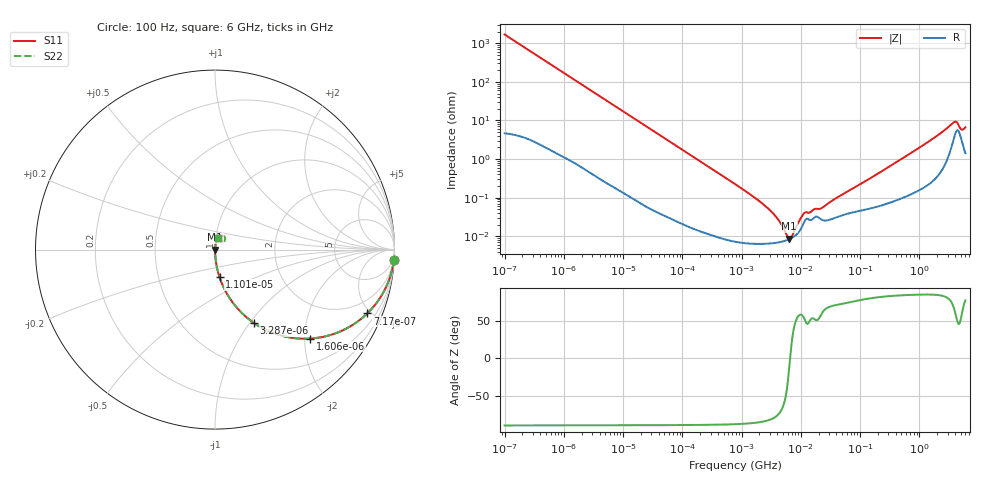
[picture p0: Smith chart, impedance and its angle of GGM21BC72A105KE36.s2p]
!Murata Part Number: GGM21BC72A105KE36
!These Parameters are Measured in Series Mode Connection
!Data Generated on Mar 13, 2026
!  o--ll--o
!Port1  Port2
!  o------o
!Operation Temp=25[degC], DC Bias Voltage=0[V]
!Freq. Start=100[Hz] Stop=6[GHz] 401[Steps]
# Hz S RI R 50
!Freq.(Hz) S11(Real) S11(Imag) S21(Real) S21(Imag) S12(Real) S12(Imag) S22(Real) S22(Imag)
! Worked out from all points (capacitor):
!   401 points, 100 Hz to 6 GHz, reference 50 ohm
!   read as one part in series: C = 938 nF near 109 Hz
!   lowest |Z| = 8.58 mohm at 6.353 MHz (marker M1)
!   series resonance near 6.592 MHz, so ESL is about 620 pH
!   S11 on the Smith chart (normalised r, x): 100 Hz: 1, -34; 717 Hz: 1.03, -4.76; 1.606 kHz: 1.01, -2.13; 3.287 kHz: 1.01, -1.05; 11.01 kHz: 1.00, -0.31; 6 GHz: 1.03, +0.13
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100  0.9964 -0.0588  0.00363 0.0588  0.00363 0.0588  0.9964 -0.0588
335  0.9618 -0.1892  0.0382 0.1892  0.0382 0.1892  0.9618 -0.1892
717  0.8484 -0.3556  0.1516 0.3556  0.1516 0.3556  0.8484 -0.3556
1606  0.532 -0.4955  0.468 0.4955  0.468 0.4955  0.532 -0.4955
2008  0.4221 -0.4904  0.5779 0.4904  0.5779 0.4904  0.4221 -0.4904
3287  0.2163 -0.4082  0.7837 0.4082  0.7837 0.4082  0.2163 -0.4082
11009  0.0252 -0.1528  0.9748 0.1528  0.9748 0.1528  0.0252 -0.1528
40335  0.00224 -0.043  0.9978 0.043  0.9978 0.043  0.00224 -0.043
774597  7.68e-05 -0.00225  0.9999 0.00225  0.9999 0.00225  7.68e-05 -0.00225
2967816  6.48e-05 -0.000478  0.9999 0.000478  0.9999 0.000478  6.48e-05 -0.000478
4060267  6.85e-05 -0.000274  0.9999 0.000274  0.9999 0.000274  6.85e-05 -0.000274
5554849  7.69e-05 -9.45e-05  0.9999 9.45e-05  0.9999 9.45e-05  7.69e-05 -9.45e-05
6353432  8.33e-05 -2.04e-05  0.9999 2.04e-05  0.9999 2.04e-05  8.33e-05 -2.04e-05
7266822  9.27e-05 5.49e-05  0.9999 -5.49e-05  0.9999 -5.49e-05  9.27e-05 5.49e-05
1.087309e7  0.000198 0.000302  0.9998 -0.000302  0.9998 -0.000302  0.000198 0.000302
1.555665e7  0.000271 0.00037  0.9997 -0.00037  0.9997 -0.00037  0.000271 0.00037
2.327686e7  0.000262 0.000488  0.9997 -0.000488  0.9997 -0.000488  0.000262 0.000488
3.124326e8  0.000769 0.00635  0.9992 -0.00635  0.9992 -0.00635  0.000769 0.00635
3.666503e9  0.032 0.0767  0.968 -0.0767  0.968 -0.0767  0.032 0.0767
4.193612e9  0.0544 0.0689  0.9456 -0.0689  0.9456 -0.0689  0.0544 0.0689
5.245841e9  0.0299 0.047  0.9701 -0.047  0.9701 -0.047  0.0299 0.047
6e9  0.018 0.0632  0.982 -0.0632  0.982 -0.0632  0.018 0.0632
